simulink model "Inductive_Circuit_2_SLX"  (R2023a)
settings: Solver=ode23s  StartTime=0.0  StopTime=10.0  MaxStep=0.001  RelTol=1e-3
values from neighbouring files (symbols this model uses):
  I_3_0 = 0*A    (= 0)    [Inductive_Circuit_2_SLX_m.m]    (also in Electric_Circuit_08_SLX_m.m; Electric_Circuit_10_SLX_m.m)
  I_5_0 = 0*A    (= 0)    [Inductive_Circuit_2_SLX_m.m]    (also in BIG_EC_Simscape_SLX_m.m; Electric_Circuit_01_SLX_m.m; Electric_Circuit_06_SLX_m.m; Electric_Circuit_09_SLX_m.m)
  I_7_0 = 0*A    (= 0)    [Inductive_Circuit_2_SLX_m.m]    (also in Electric_Circuit_01_SLX_m.m; Electric_Circuit_09_SLX_m.m)
  I_8_0 = 0*A    (= 0)    [Inductive_Circuit_2_SLX_m.m]    (also in Electric_Circuit_02_SLX_m.m; Electric_Circuit_05_SLX_m.m; Electric_Circuit_06_SLX_m.m; Electric_Circuit_07_SLX_m.m)
  L_3 = 0.002*H    (= 0.002)    [Inductive_Circuit_2_EQN.m]    (also in Inductive_Circuit_2_SLX_m.m; Electric_Circuit_08_EQN.m; Electric_Circuit_08_SLX_m.m; Electric_Circuit_10_EQN.m)
  L_5 = 0.002*H    (= 0.002)    [Inductive_Circuit_2_EQN.m]    (also in Inductive_Circuit_2_SLX_m.m; BIG_EC_Simscape_EQN.m; BIG_EC_Simscape_SLX_m.m; Electric_Circuit_01_EQN.m)
  L_7 = 0.002*H    (= 0.002)    [Inductive_Circuit_2_EQN.m]    (also in Inductive_Circuit_2_SLX_m.m; Electric_Circuit_09_EQN.m; Electric_Circuit_09_SLX_m.m)
  R_2 = 100*Ohm    (= 100)    [Inductive_Circuit_2_EQN.m]    (also in Inductive_Circuit_2_SLX_m.m; BIG_EC_Simscape_EQN.m; BIG_EC_Simscape_SLX_m.m; Electric_Circuit_07_EQN.m)
  R_4 = 100*Ohm    (= 100)    [Inductive_Circuit_2_EQN.m]    (also in Inductive_Circuit_2_SLX_m.m; BIG_EC_Simscape_EQN.m; BIG_EC_Simscape_SLX_m.m; Electric_Circuit_08_EQN.m)
  R_6 = 100*Ohm    (= 100)    [Inductive_Circuit_2_EQN.m]    (also in Inductive_Circuit_2_SLX_m.m; BIG_EC_Simscape_EQN.m; BIG_EC_Simscape_SLX_m.m; Electric_Circuit_02_EQN.m)
  Ts = Tfin/Nr_Ts_Points    (= 1.9482e-07)    [Inductive_Circuit_2_SLX_m.m]    (also in BIG_EC_Simscape_SLX_m.m = 0.0003; Car_Dumper_SLX_m.m = 0.0022779; Electric_Circuit_01_SLX_m.m = 0.005; Electric_Circuit_02_SLX_m.m = 0.000480145)
  V_1_0 = 10*V    (= 10)    [Inductive_Circuit_2_SLX_m.m]    (also in BIG_EC_Simscape_SLX_m.m; Electric_Circuit_02_SLX_m.m; Electric_Circuit_03_SLX_m.m; Electric_Circuit_04_SLX_m.m)

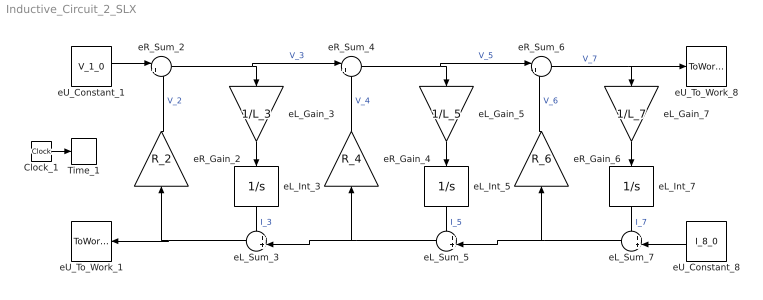
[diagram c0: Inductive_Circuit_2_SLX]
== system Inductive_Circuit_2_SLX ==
  Clock_1 : Clock
  Time_1 : ToWorkspace  VariableName=t  SaveFormat=Timeseries  SampleTime=Ts
  eL_Gain_3 : Gain  Gain=1/L_3  Multiplication=Matrix(K*u)
  eL_Gain_5 : Gain  Gain=1/L_5  Multiplication=Matrix(K*u)
  eL_Gain_7 : Gain  Gain=1/L_7  Multiplication=Matrix(K*u)
  eL_Int_3 : Integrator  InitialCondition=I_3_0
  eL_Int_5 : Integrator  InitialCondition=I_5_0
  eL_Int_7 : Integrator  InitialCondition=I_7_0
  eL_Sum_3 : Sum  Inputs=++|
  eL_Sum_5 : Sum  Inputs=++|
  eL_Sum_7 : Sum  Inputs=++|
  eR_Gain_2 : Gain  Gain=R_2  Multiplication=Matrix(K*u)
  eR_Gain_4 : Gain  Gain=R_4  Multiplication=Matrix(K*u)
  eR_Gain_6 : Gain  Gain=R_6  Multiplication=Matrix(K*u)
  eR_Sum_2 : Sum  Inputs=|+-
  eR_Sum_4 : Sum  Inputs=|+-
  eR_Sum_6 : Sum  Inputs=|+-
  eU_Constant_1 : Constant  Value=V_1_0
  eU_Constant_8 : Constant  Value=I_8_0
  eU_To_Work_1 : ToWorkspace  VariableName=I_1_0  SaveFormat=Timeseries  SampleTime=Ts
  eU_To_Work_8 : ToWorkspace  VariableName=V_8_0  SaveFormat=Timeseries  SampleTime=Ts
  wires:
  eU_Constant_1/1 -> eR_Sum_2/1
  eR_Sum_2/1 -> eL_Gain_3/1, eR_Sum_4/1  "V_3"
  eL_Sum_3/1 -> eU_To_Work_1/1, eR_Gain_2/1
  eR_Gain_2/1 -> eR_Sum_2/2  "V_2"
  eL_Sum_5/1 -> eL_Sum_3/2, eR_Gain_4/1
  eL_Gain_3/1 -> eL_Int_3/1
  eL_Int_3/1 -> eL_Sum_3/1  "I_3"
  eR_Sum_4/1 -> eL_Gain_5/1, eR_Sum_6/1  "V_5"
  eR_Gain_4/1 -> eR_Sum_4/2  "V_4"
  eL_Sum_7/1 -> eL_Sum_5/2, eR_Gain_6/1
  eL_Gain_5/1 -> eL_Int_5/1
  eL_Int_5/1 -> eL_Sum_5/1  "I_5"
  eR_Sum_6/1 -> eU_To_Work_8/1, eL_Gain_7/1  "V_7"
  eR_Gain_6/1 -> eR_Sum_6/2  "V_6"
  eU_Constant_8/1 -> eL_Sum_7/2
  eL_Gain_7/1 -> eL_Int_7/1
  eL_Int_7/1 -> eL_Sum_7/1  "I_7"
  Clock_1/1 -> Time_1/1
